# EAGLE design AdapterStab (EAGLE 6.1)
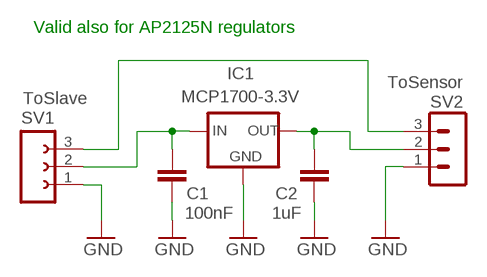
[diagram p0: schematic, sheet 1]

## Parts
C1  100nF  C-EUC0805  [C0805]
C2  1uF  C-EUC0805  [C0805]
IC1  MCP1700-3.3V  MCP1700SOT23  [SOT23]
SV1  ToSlave  FE03-1"  [FE03-1]
SV2  ToSensor  MA03-1N  [MA03-1]

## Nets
GND: C1.2 C2.2 IC1.1(GND) SV1.1 SV2.1
N$1: C1.1 IC1.3(IN) SV1.2
N$2: C2.1 IC1.2(OUT) SV2.2
N$3: SV1.3 SV2.3

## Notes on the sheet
- Valid also for AP2125N regulators

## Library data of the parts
C1 C2 = 00-LIVIO:C-EU: CAPACITOR, European symbol
IC1 = 00-LIVIO:MCP1700: Linear regulator Quescient courrent 1.8uA Input 2.3v to 6v Output 1.2v 1.8v 2.5v 3.0v 3.3v 5.0v
SV1 = 02-con-lsta-F:FE03-1: FEMALE HEADER
SV2 = 03-con-lstb-M:MA03-1: PIN HEADER

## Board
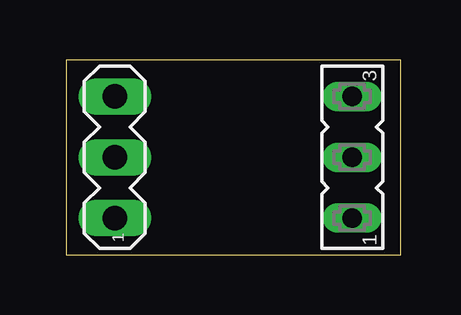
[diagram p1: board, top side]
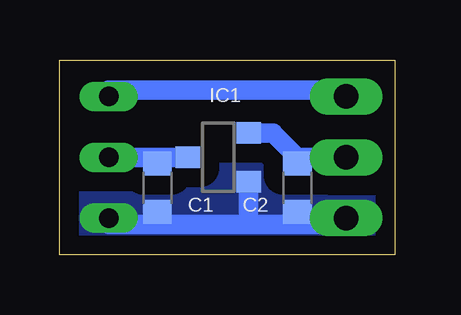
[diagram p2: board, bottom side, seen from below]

Size 13.97 x 8.13 mm. Coordinates in mm from the lower left corner, seen from the top.
Outline: 13.97,8.13 0,8.13 0,0 13.97,0 13.97,8.13
Copper layers (1*16): Top 0.035mm / dielectric 1.5mm / Bottom 0.035mm
Design rules: minimum track width 10mil, minimum drill 0.6mm, track to track 8mil, track to pad 8mil, pad to pad 8mil, via to via 8mil, smd to smd 8mil, copper to edge 31mil, drill to drill 8mil, minimum pad ring 5mil, minimum via ring 8mil, stop-mask expansion 4mil, vias tented up to drill 0mil, thermal gap 41mil

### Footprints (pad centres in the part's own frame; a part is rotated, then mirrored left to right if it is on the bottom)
C0805 = smd 1 x 1.2: 1 -1.016,0; 2 1.016,0
SOT23 = smd 0.889 x 1.016: 1 -1.016,-1.27; 2 1.016,-1.27; 3 0,1.27
FE03-1 = drill 0.813 long: 1 -2.54,0; 2 0,0; 3 2.54,0
MA03-1 = drill 1.016 long: 1 -2.54,0; 2 0,0; 3 2.54,0

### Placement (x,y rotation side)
C1  9.91,2.79 270 bottom
C2  4.06,2.79 270 bottom
IC1  7.37,4.06 90 bottom
SV1  11.94,4.06 90 top
SV2  2.03,4.06 90 top

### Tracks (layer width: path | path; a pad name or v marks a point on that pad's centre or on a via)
GND
  Bottom 0.813: 6.1,1.27 9.91,1.27 | 4.06,1.27 6.1,1.27 | 4.06,1.27 2.29,1.27 SV2.1 | 9.91,1.27 C1.2 | 6.1,1.27 IC1.1 | 4.06,1.27 C2.2 | 9.91,1.27 11.94,1.27 SV1.1
  pour Bottom (isolate 0.8, rank 6, no thermals): -1,-1 14.97,-1 14.97,9.13 -1,9.13
N$1
  Bottom 0.813: 9.91,4.06 C1.1 9.91,4.06 | 9.91,4.06 IC1.3 | 9.91,4.06 SV1.2
N$2
  Bottom 0.813: IC1.2 5.08,5.08 4.06,4.06 | 4.06,4.06 C2.1 4.06,4.06 | 4.06,4.06 3.3,4.06 SV2.2
N$3
  Bottom 0.813: SV2.3 2.29,6.86 11.94,6.86 SV1.3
